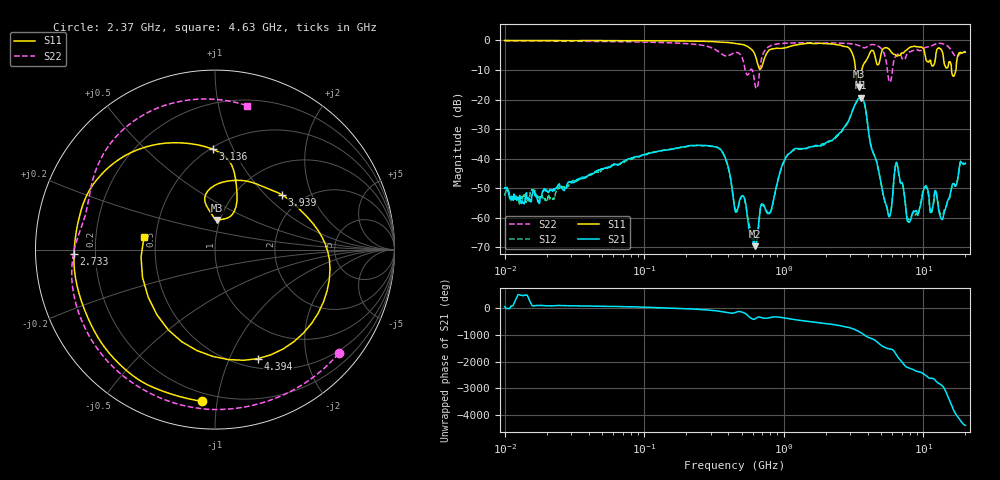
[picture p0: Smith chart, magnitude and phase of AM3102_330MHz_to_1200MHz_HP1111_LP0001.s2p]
! Date/Time: Tue, Sep 11, 2018 5:24 PM
! Network Analyzer: Agilent Technologies E8362B Rev: A.07.50.63
! Sweep from 0.010 to 20.000 GHz, 1601 Points, Sweep Type: LOG
! Power Supply: 4.949 V, 0.001 A
# Hz S DB R 50
!freq MagS11 AngS11 MagS21 AngS21 MagS12 AngS12 MagS22 AngS22
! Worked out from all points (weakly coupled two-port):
!   1601 points, 10 MHz to 20 GHz, reference 50 ohm
!   highest |S21| = -19.36 dB at 3.549 GHz (marker M1); lowest = -69.6 dB at 623.6 MHz (marker M2)
!   lowest |S11| = -15.7 dB at 3.449 GHz (marker M3), VSWR 1.39, Z = 48.4 + j16.4 ohm
!   |S11| at or under -10 dB: 3.266 GHz to 3.62 GHz (354.2 MHz wide, 10.3 % of centre); 15.91 GHz to 17.11 GHz (1.2 GHz wide, 7.27 % of centre)
!   |S22| runs from -16.2 to -0.2 dB; largest |S21 - S12| = 0.0059
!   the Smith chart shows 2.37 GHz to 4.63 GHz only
!   S11 on the Smith chart (normalised r, x): 2.37 GHz: 0.15, -0.91; 2.733 GHz: 0.12, -0.02; 3.136 GHz: 0.51, +0.84; 3.939 GHz: 1.58, +1.26; 4.394 GHz: 0.61, -1.28; 4.63 GHz: 0.43, +0.07
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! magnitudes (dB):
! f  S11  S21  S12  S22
! 10 MHz  0.0  -50.0  -52.6  -0.2
! 35.55 MHz  -0.1  -46.8  -46.4  -0.3
! 126.4 MHz  -0.2  -37.5  -37.5  -0.7
! 344.4 MHz  -0.6  -36.6  -36.5  -4.0
! 447.2 MHz  -1.0  -57.5  -56.8  -4.1
! 623.6 MHz  -5.0  -69.6  -69.4  -15.3
! 1.037 GHz  -2.5  -39.5  -39.5  -0.9
! 1.59 GHz  -1.1  -36.0  -35.9  -0.8
! 2.37 GHz  -1.4  -32.4  -32.8  -0.9
! 2.733 GHz  -2.1  -29.2  -29.5  -1.0
! 3.136 GHz  -5.0  -23.3  -23.4  -1.2
! 3.449 GHz  -15.7  -19.7  -19.7  -1.7
! 3.549 GHz  -12.8  -19.4  -19.3  -2.0
! 3.939 GHz  -6.3  -26.3  -26.3  -2.2
! 4.394 GHz  -3.7  -38.3  -38.2  -1.4
! 4.63 GHz  -7.9  -41.1  -41.2  -1.7
! 5.652 GHz  -2.9  -59.6  -59.3  -13.5
! 6.426 GHz  -5.3  -41.2  -41.6  -4.9
! 7.882 GHz  -2.6  -61.5  -60.6  -4.0
! 10.38 GHz  -5.9  -49.2  -49.5  -2.4
! 13.68 GHz  -3.9  -60.6  -59.1  -1.1
! 20 GHz  -3.9  -41.5  -41.9  -3.8
